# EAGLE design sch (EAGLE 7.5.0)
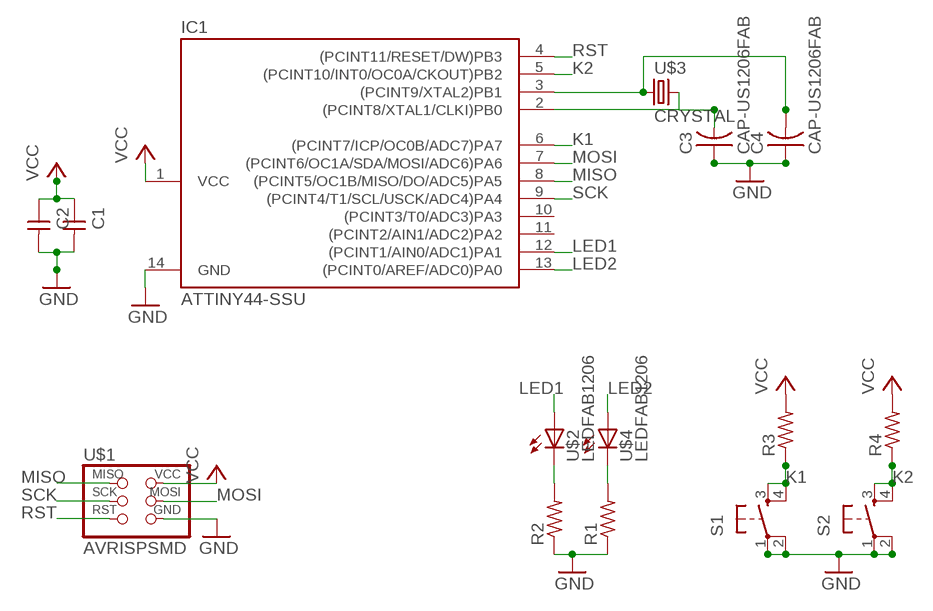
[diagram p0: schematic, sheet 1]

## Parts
C1  CAP-UNPOLARIZEDFAB  [C1206FAB]
C2  CAP-UNPOLARIZEDFAB  [C1206FAB]
C3  CAP-US1206FAB  [C1206FAB]
C4  CAP-US1206FAB  [C1206FAB]
IC1  ATTINY44-SSU  [SOIC14]
R1  RES-US1206FAB  [R1206FAB]
R2  RES-US1206FAB  [R1206FAB]
R3  RES-US1206FAB  [R1206FAB]
R4  RES-US1206FAB  [R1206FAB]
S1  6MM_SWITCH6MM_SWITCH  [6MM_SWITCH]
S2  6MM_SWITCH6MM_SWITCH  [6MM_SWITCH]
U$1  AVRISPSMD  [2X03SMD]
U$2  LEDFAB1206  [LED1206FAB]
U$3  CRYSTAL  [2-SMD-5X3MM]
U$4  LEDFAB1206  [LED1206FAB]

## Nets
GND: C1.2 C2.2 C3.1 C4.1 IC1.14(GND) R1.1 R2.1 S1.1(P) S1.2(P1) S2.1(P) S2.2(P1) U$1.6(GND)
K1: IC1.6((PCINT7/ICP/OC0B/ADC7)PA7) R3.1 S1.3(S) S1.4(S1)
K2: IC1.5((PCINT10/INT0/OC0A/CKOUT)PB2) R4.1 S2.3(S) S2.4(S1)
LED1: IC1.12((PCINT1/AIN0/ADC1)PA1) U$2.1(A)
LED2: IC1.13((PCINT0/AREF/ADC0)PA0) U$4.1(A)
MISO: IC1.8((PCINT5/OC1B/MISO/DO/ADC5)PA5) U$1.1(MISO)
MOSI: IC1.7((PCINT6/OC1A/SDA/MOSI/ADC6)PA6) U$1.4(MOSI)
N$1: R1.2 U$4.2(C)
N$2: R2.2 U$2.2(C)
N$3: C4.2 IC1.3((PCINT9/XTAL2)PB1) U$3.P$1
N$5: C3.2 IC1.2((PCINT8/XTAL1/CLKI)PB0) U$3.P$2
RST: IC1.4((PCINT11/RESET/DW)PB3) U$1.5(RST)
SCK: IC1.9((PCINT4/T1/SCL/USCK/ADC4)PA4) U$1.3(SCK)
VCC: C1.1 C2.1 IC1.1(VCC) R3.2 R4.2 U$1.2(VCC)
Unconnected: IC1.10((PCINT3/T0/ADC3)PA3) IC1.11((PCINT2/AIN1/ADC2)PA2)

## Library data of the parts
C1 C2 = fab:CAP-UNPOLARIZED
C3 C4 = fab:CAP-US
IC1 = fab:ATTINY44
R1-R4 = fab:RES-US: Resistor (US Symbol)
S1 S2 = fab:6MM_SWITCH: OMRON SWITCH
U$1 = fab:AVRISP
U$2 U$4 = fab:LED: LED
U$3 = fab:CRYSTAL

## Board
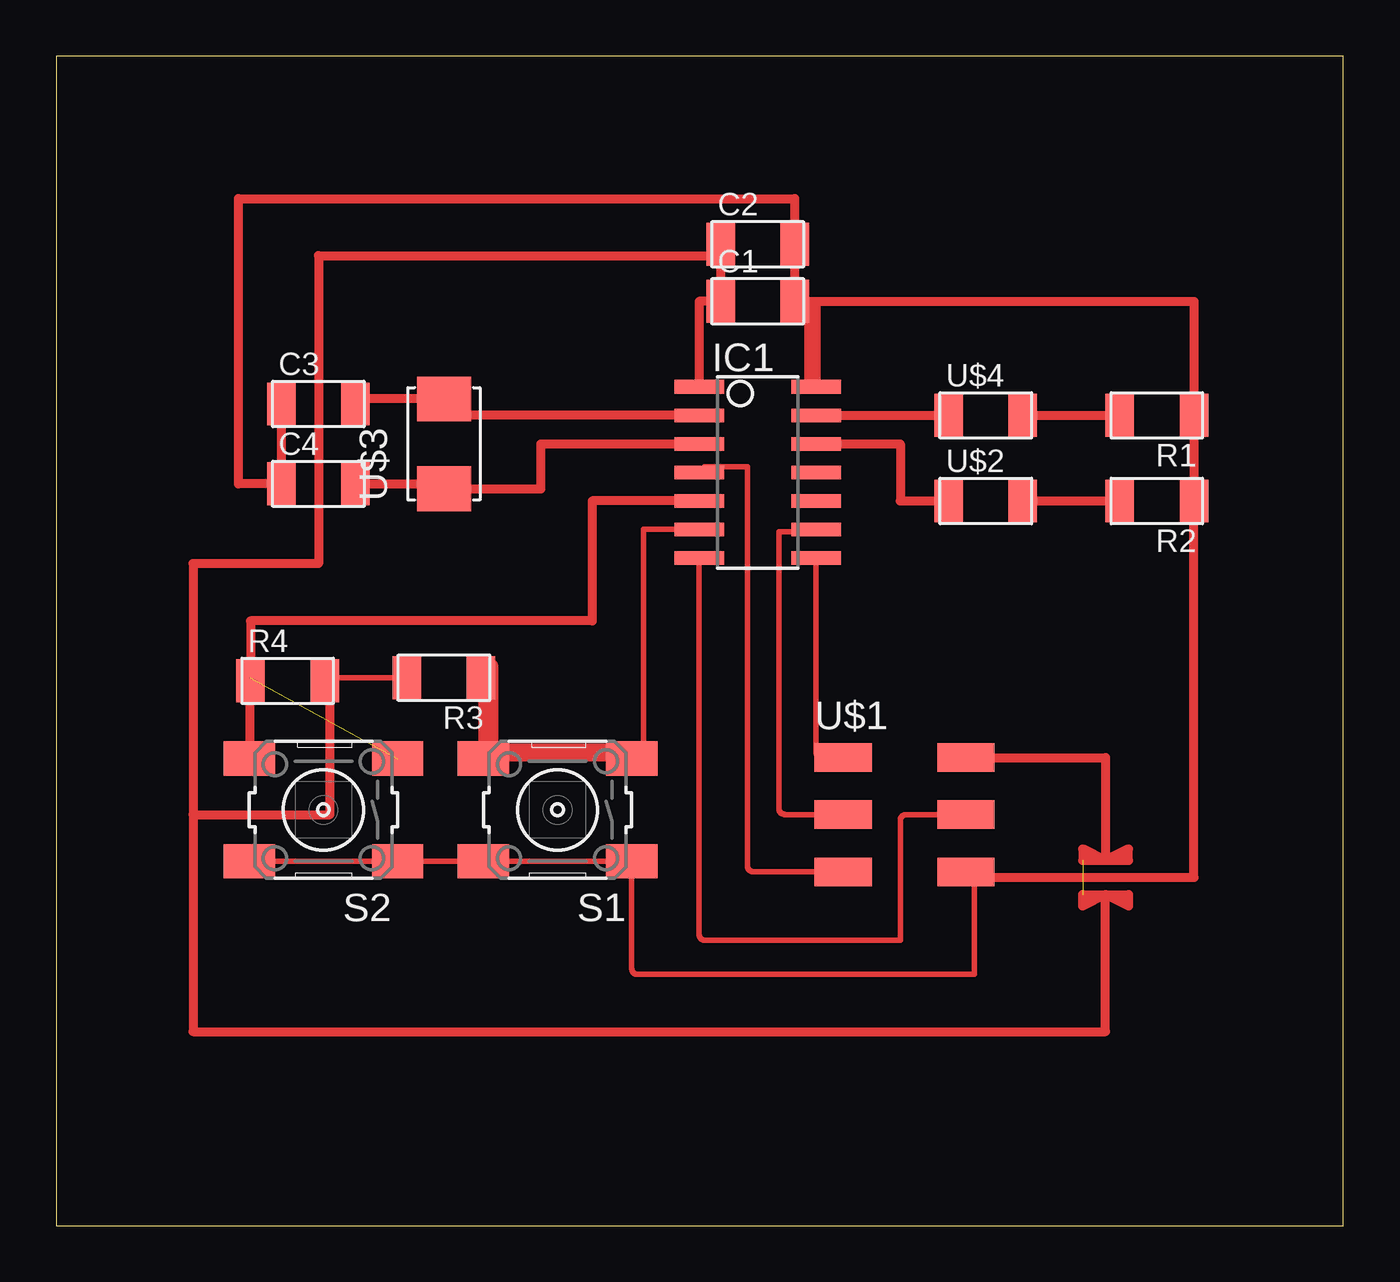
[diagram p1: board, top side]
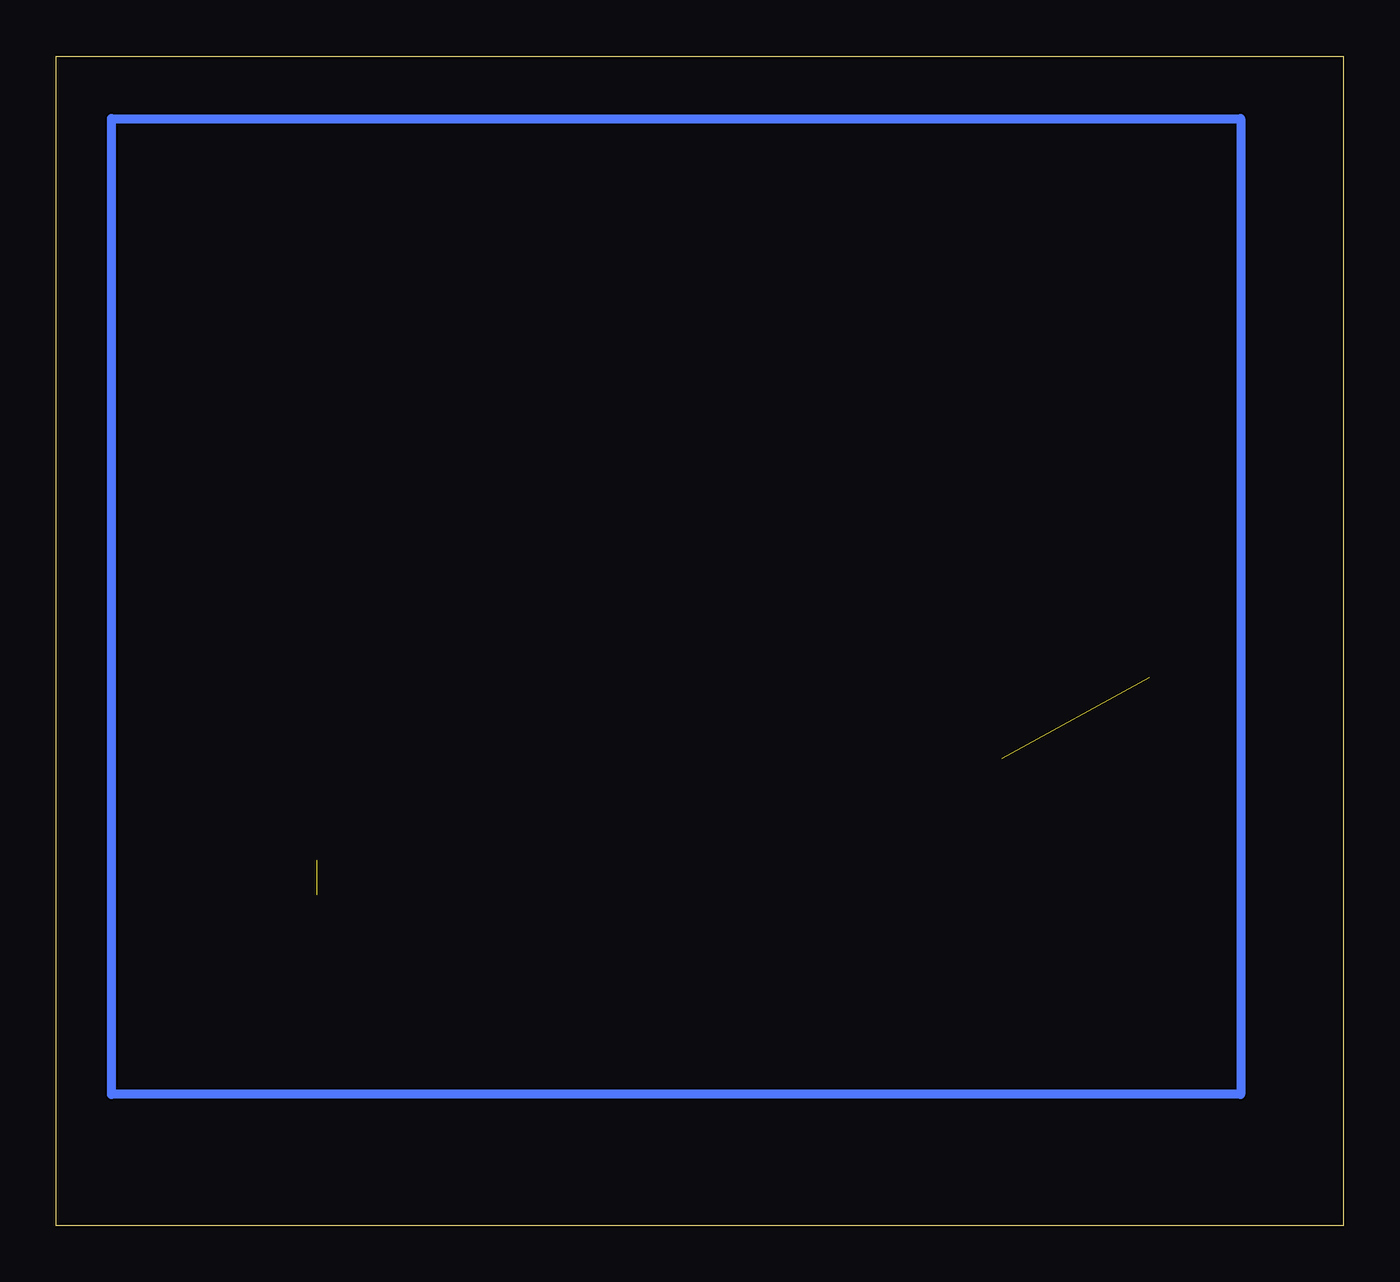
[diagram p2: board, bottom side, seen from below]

Size 57.33 x 52.06 mm. Coordinates in mm from the lower left corner, seen from the top.
Outline: 0,0 57.33,0 57.33,52.06 0,52.06 0,0
Copper layers (1*16): Top 0.035mm / dielectric 1.5mm / Bottom 0.035mm
Design rules "default": minimum track width 10mil, minimum drill 24mil, track to track 8mil, track to pad 8mil, pad to pad 8mil, via to via 8mil, smd to smd 8mil, copper to edge 40mil, drill to drill 8mil, minimum pad ring 10mil, minimum via ring 8mil, stop-mask expansion 4mil, vias tented up to drill 0mil, thermal gap 10mil

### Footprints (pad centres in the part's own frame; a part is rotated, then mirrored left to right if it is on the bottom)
C1206FAB = smd 1.27 x 1.905: 1 -1.651,0; 2 1.651,0
SOIC14 = smd 0.61 x 2.21: 1 -3.81,-2.603; 2 -2.54,-2.603; 3 -1.27,-2.603; 4 0,-2.603; 5 1.27,-2.603; 6 2.54,-2.603; 7 3.81,-2.603; 8 3.81,2.603; 9 2.54,2.603; 10 1.27,2.603; 11 0,2.603; 12 -1.27,2.603; 13 -2.54,2.603; 14 -3.81,2.603
R1206FAB = smd 1.27 x 1.905: 1 -1.651,0; 2 1.651,0
6MM_SWITCH = smd 2.286 x 1.524: 1 -3.302,2.286; 2 3.302,2.286; 3 -3.302,-2.286; 4 3.302,-2.286
2X03SMD = smd 2.54 x 1.27: 1 -2.54,2.54; 2 2.92,2.54; 3 -2.54,0; 4 2.92,0; 5 -2.54,-2.54; 6 2.92,-2.54
LED1206FAB = smd 1.27 x 1.905: 1 -1.651,0; 2 1.651,0
2-SMD-5X3MM = smd 2 x 2.4: P$1 -2,0; P$2 2,0

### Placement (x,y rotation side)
C1  31.24,41.15 0 top
C2  31.24,43.69 0 top
C3  11.68,36.58 0 top
C4  11.68,33.02 0 top
IC1  31.24,33.53 270 top
R1  49.02,36.07 180 top
R2  49.02,32.26 180 top
R3  17.27,24.38 180 top
R4  10.31,24.25 0 top
S1  22.33,18.5 180 top
S2  11.9,18.5 180 top
U$1  37.59,18.29 0 top
U$2  41.4,32.26 0 top
U$3  17.27,34.8 90 top
U$4  41.4,36.07 0 top

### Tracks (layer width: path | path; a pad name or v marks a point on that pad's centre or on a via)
GND
  Top 0.254: U$1.6 40.64,15.75 arc-90 40.89,15.49 40.89,11.18 25.89,11.18 arc-90 25.64,11.43 S1.1 S1.2 S2.1 arc90 S2.1 S2.2
  Top 0.406: C3.1 C4.1 8.13,33.02 8.13,45.72 32.89,45.72 C2.2 C1.2 33.53,41.15 | 40.89,15.49 50.67,15.49 R2.1 R1.1 50.67,41.15 33.85,41.15 | 33.53,41.15 33.85,41.15 | 33.85,41.15 IC1.14 33.53,37.34 33.53,41.15
K1
  Top 0.254: IC1.6 26.16,30.99 26.16,21.05 arc-90 25.91,20.79 S1.3 S1.4 arc-90 18.92,20.9 R3.1
K2  (1 unrouted)
  Top 0.254: R4.1 arc90 8.6,24.19 S2.4
  Top 0.406: IC1.5 23.88,32.26 23.88,26.92 8.66,26.92 R4.1 | S2.4 8.64,20.79 8.64,24.38
LED1
  Top 0.406: IC1.12 37.59,34.8 37.59,32.26 U$2.1
LED2
  Top 0.406: IC1.13 U$4.1
MISO
  Top 0.254: U$1.1 34.1,20.83 arc-90 33.85,21.08 IC1.8
MOSI
  Top 0.254: U$1.4 37.85,18.29 arc90 37.59,18.03 37.59,12.7 28.89,12.7 arc-90 28.64,12.95 IC1.7
N$1
  Top 0.406: U$4.2 R1.2 47.75,36.07
N$2
  Top 0.406: U$2.2 R2.2
N$3
  Top 0.406: IC1.3 21.59,34.8 21.59,32.8 U$3.P$1 17.27,33.02 C4.2
N$4
  Bottom 0.406: 4.57,49.28 4.57,5.84 54.86,5.84 54.86,49.28 4.57,49.28
N$5
  Top 0.406: IC1.2 17.27,36.07 U$3.P$2 13.34,36.8 C3.2
RST
  Top 0.254: U$1.5 31.05,15.75 arc-90 30.8,16 30.8,33.79 28.89,33.79 arc-90 IC1.4
S$3
  Top 0.762: 19.3,24.89 19.3,21.08 25.4,21.08
SCK
  Top 0.254: U$1.3 32.46,18.29 arc-90 32.44,18.31 arc-90 32.19,18.56 32.19,30.89 33.75,30.89 arc90 IC1.9
VCC  (1 unrouted)
  Top 0.254: R3.2 12.1,24.38 arc90 R4.2
  Top 0.406: 28.45,37.34 IC1.1 28.64,41.15 C1.1 29.59,43.18 | 6.1,18.29 6.1,29.46 11.68,29.46 11.68,43.18 29.59,43.18 | 6.1,18.29 12.19,18.29 12.19,23.88 11.96,23.88 R4.2 | 6.1,18.29 6.1,8.64 46.74,8.64 46.74,14.73 | U$1.2 46.74,20.83 46.74,16.26 | 46.74,16.26 45.72,16.76 45.72,16.26 46.74,16.26 | 46.74,16.26 47.75,16.26 47.75,16.76 46.74,16.26 | 46.74,14.73 45.72,14.73 45.72,14.22 46.74,14.73 | 46.74,14.73 47.75,14.73 47.75,14.22 46.74,14.73 | 29.59,43.18 C2.1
